[IBIS Ver]   3.2
[File Name]   sprm144.ibs
[File Rev]   0.3
[Date]   March 17, 2003
[Source]   IBIS Model Generated from PACED 4.51D
[Disclaimer]   Please be aware that in the absence of a written agreement
|   Texas Instruments(TI) assumes no liability for:
|   (1) The accuracy of the IBIS models provided to your company
|   (2) The proper functioning of these Models in your design
|   or for any resulting applications; or
|   (3)Infringement of patents, copyrights or intellectual
|   property rights resulting from your use of these models.
|   TI provides IBIS Models as a service to our customers and
|   therefore reserves the right to limit distribution of the
|   Models.
[Copyright]   Property of Texas Instruments Incorporated.
|   Unauthorized reproduction and/or distribution is strictly.
|   prohibited.
|   This product is protected under copyright law and trade
|   secret law as an unpublished work.
|   Created 2002,(C) Copyright 2002,
|   Texas Instruments Incorporated., All Rights Reserved.
|   These commodities are under the U.S.
|   Government distribution license control. As such,they are
|   not to be re-exported without the prior approval of the U.S.
|   Department of Commerce.
[Notes]   Revision History
|   0.3  Updated CLKOUT3 buffer to reflect silicon revision 2.0
|   for C6712D GDP device.
[Component]   c6712d_GDP
[Manufacturer]   Texas Instruments
[Package]
| Variable   Typ   Min   Max
R_pkg   0.15798   0.1249   0.19129
L_pkg   4.816e-09   3.586e-09   6.029e-09
C_pkg   1.362e-12   8.298e-13   1.789e-12
[Pin] signal_name   model_name   R_pin   L_pin   C_pin
A3   CLKIN   IDH091PE1001   0.18019   5.664E-09   1.7625E-12
Y12   CLKOUT2/GP2   IDH091UOS335PE1001  0.16709   5.124E-09   1.4203E-12
D10   CLKOUT3   OUK831PE1001   0.12485   3.586E-09   9.165E-13
C4   CLKMODE0   IDH091PS1001   0.15399   4.656E-09   1.3457E-12
B7   TMS   IDH091PS1001   0.15672   4.757E-09   1.3298E-12
A8   TDO   OUK831PS1001   0.16876   5.201E-09   1.4526E-12
A7   TDI   IDH091PS1001   0.17187   5.326E-09   1.4901E-12
A6   TCK   IDH091PS1001   0.17452   5.436E-09   1.563E-12
B6   TRSTz   IDH091PE1001   0.15745   4.805E-09   1.3514E-12
B12   EMU5   IDH091OUK831PS1001  0.1503   4.526E-09   1.2197E-12
C11   EMU4   IDH091OUK831PS1001  0.13457   3.948E-09   1.034E-12
B10   EMU3   IDH091OUK831PS1001  0.14073   4.347E-09   1.3521E-12
D3   EMU2   IDH091OUK831PS1001  0.15496   4.735E-09   1.2636E-12
B9   EMU1   IDH091OUK831PS1001  0.15386   4.643E-09   1.2548E-12
D9   EMU0   IDH091OUK831PS1001  0.12688   3.663E-09   9.161E-13
A13   RESETz   IDG091PS1001   0.1637   5.019E-09   1.3754E-12
C13   NMI   IDH091PE1001   0.139   4.115E-09   1.1233E-12
E3   GP7   IDH091OUK831PS1001  0.14773   4.469E-09   1.2867E-12
D2   GP6   IDH091OUK831PS1001  0.16895   5.218E-09   1.4683E-12
C1   GP5   IDH091OUK831PS1001  0.17903   5.639E-09   1.7233E-12
C2   GP4   IDH091OUK831PS1001  0.15766   4.795E-09   1.383E-12
V6   CE3z   IDH091OUK831PS1001  0.14621   4.39E-09   1.2151E-12
W6   CE2z   IDH091OUK831PS1001  0.16098   4.921E-09   1.4132E-12
W18   CE1z   IDH091OUK831PS1001  0.17556   5.446E-09   1.6489E-12
V17   CE0z   IDH091OUK831PS1001  0.15744   4.8E-09   1.3798E-12
U19   BE1z   IDH091OUK831PS1001  0.16093   4.997E-09   1.4815E-12
V20   BE0z   IDH091OUK831PS1001  0.17611   5.497E-09   1.6313E-12
J18   HOLDAz   IDH091OUK831PS1001  0.14188   4.206E-09   1.1141E-12
J17   HOLDz   IDH091OUK831PS1001  0.13083   3.807E-09   9.644E-13
J19   BUSREQ   IDH091OUK831PS1001  0.14582   4.359E-09   1.1679E-12
Y11   ECLKIN   IDH091PE1001   0.16208   0.000000005   1.4122E-12
Y10   ECLKOUT   UOS335PE1001   0.16106   4.931E-09   1.345E-12
V11   SDCASz   IDH091OUK831PS1001  0.1364   4.059E-09   1.03E-12
W10   SDRASz   IDH091OUK831PS1001  0.1486   4.45E-09   1.1911E-12
V12   SDWEz   IDH091OUK831PS1001  0.14012   4.139E-09   1.0969E-12
Y5   ARDY   IDH091OUK831PS1001  0.17592   5.451E-09   1.6354E-12
U18   EA21   IDH091OUK831PS1001  0.13802   4.156E-09   1.129E-12
Y18   EA20   IDH091OUK831PS1001  0.18588   5.849E-09   1.7404E-12
W17   EA19   IDH091OUK831PS1001  0.16927   5.225E-09   1.5492E-12
Y16   EA18   IDH091OUK831PS1001  0.17911   5.584E-09   1.6036E-12
V16   EA17   IDH091OUK831PS1001  0.15217   4.613E-09   1.3114E-12
Y15   EA16   IDH091OUK831PS1001  0.17574   5.447E-09   1.5678E-12
W15   EA15   IDH091OUK831PS1001  0.16072   4.894E-09   1.4026E-12
Y14   EA14   IDH091OUK831PS1001  0.1722   5.313E-09   1.5193E-12
W14   EA13   IDH091OUK831PS1001  0.15855   4.806E-09   1.3767E-12
V14   EA12   IDH091OUK831PS1001  0.14298   4.247E-09   1.1833E-12
W13   EA11   IDH091OUK831PS1001  0.15509   4.674E-09   1.3133E-12
V10   EA10   IDH091OUK831PS1001  0.1353   3.969E-09   1.0187E-12
Y9   EA9   IDH091OUK831PS1001  0.1646   5.033E-09   1.4055E-12
V9   EA8   IDH091OUK831PS1001  0.13792   4.071E-09   1.0499E-12
Y8   EA7   IDH091OUK831PS1001  0.16615   5.125E-09   1.4253E-12
W8   EA6   IDH091OUK831PS1001  0.1525   4.599E-09   1.2789E-12
V8   EA5   IDH091OUK831PS1001  0.14065   4.164E-09   1.1235E-12
W7   EA4   IDH091OUK831PS1001  0.15712   4.787E-09   1.3445E-12
V7   EA3   IDH091OUK831PS1001  0.1433   4.261E-09   1.1748E-12
Y6   EA2   IDH091OUK831PS1001  0.17352   5.39E-09   1.5923E-12
T19   ED15   IDH091OUK831PS1001  0.16189   4.967E-09   1.4499E-12
T20   ED14   IDH091OUK831PS1001  0.17215   5.387E-09   1.5831E-12
T18   ED13   IDH091OUK831PS1001  0.15033   4.53E-09   1.3312E-12
R20   ED12   IDH091OUK831PS1001  0.17084   5.33E-09   1.5388E-12
R19   ED11   IDH091OUK831PS1001  0.15882   4.87E-09   1.3707E-12
P20   ED10   IDH091OUK831PS1001  0.16585   5.138E-09   1.4498E-12
P18   ED9   IDH091OUK831PS1001  0.14348   4.278E-09   1.1512E-12
N20   ED8   IDH091OUK831PS1001  0.16474   5.075E-09   1.4344E-12
N19   ED7   IDH091OUK831PS1001  0.15249   4.606E-09   1.2735E-12
N18   ED6   IDH091OUK831PS1001  0.1392   4.109E-09   1.0975E-12
M20   ED5   IDH091OUK831PS1001  0.16351   4.995E-09   1.4105E-12
M19   ED4   IDH091OUK831PS1001  0.15158   4.535E-09   1.2513E-12
L19   ED3   IDH091OUK831PS1001  0.15121   4.529E-09   1.2368E-12
L18   ED2   IDH091OUK831PS1001  0.13524   3.962E-09   1.023E-12
K19   ED1   IDH091OUK831PS1001  0.14992   4.542E-09   1.2211E-12
K18   ED0   IDH091OUK831PS1001  0.13736   4.069E-09   1.0426E-12
F1   TOUT1   IDH091OUK831PE1001  0.17453   5.437E-09   1.5615E-12
F2   TINP1   IDH091OUK831PE1001  0.15861   4.866E-09   1.3778E-12
G1   TOUT0   IDH091OUK831PE1001  0.16999   5.241E-09   1.5004E-12
G2   TINP0   IDH091OUK831PE1001  0.15603   4.739E-09   1.3418E-12
E1   CLKS1   IDG091UOS205   0.17483   5.458E-09   1.617E-12
M1   CLKR1   IDH091OUK831PE1001  0.16737   5.138E-09   1.4594E-12
L3   CLKX1   IDH091OUK831PE1001  0.13844   4.083E-09   1.0869E-12
M2   DR1   IDG091UOS205   0.15325   4.608E-09   1.3011E-12
L2   DX1   IDH091OUK831PS1001  0.15147   4.517E-09   1.3075E-12
M3   FSR1   IDH091OUK831PE1001  0.13992   4.134E-09   1.1163E-12
L1   FSX1   IDH091OUK831PE1001  0.16353   4.946E-09   1.4648E-12
K3   CLKS0   IDH091OUK831PE1001  0.13597   4.005E-09   1.0142E-12
H3   CLKR0   IDH091OUK831PE1001  0.13887   4.103E-09   1.1188E-12
G3   CLKX0   IDH091OUK831PE1001  0.14227   4.232E-09   1.1737E-12
J1   DR0   IDH091OUK831PS1001  0.16689   5.141E-09   1.3597E-12
H2   DX0   IDH091OUK831PS1001  0.15223   4.578E-09   1.31E-12
J3   FSR0   IDH091OUK831PE1001  0.13605   4.002E-09   1.0327E-12
H1   FSX0   IDH091OUK831PE1001  0.16688   5.126E-09   1.4562E-12
| End of package information
| Component   IDG091PS1001
[Component]   IDG091PS1001
[Manufacturer]   Texas Instruments
[Package]
|   typ   min   max
R_pkg   0   0   0
L_pkg   0   0   0
C_pkg   0   0   0
[Pin]   signal_name   model_name   R_pin   L_pin   C_pin
   1   A   IDG091PS1001   0   0   0
| Component   IDG091UOS205
[Component]   IDG091UOS205
[Manufacturer]   Texas Instruments
[Package]
|   typ   min   max
R_pkg   0   0   0
L_pkg   0   0   0
C_pkg   0   0   0
[Pin]   signal_name   model_name   R_pin   L_pin   C_pin
   1   Y   IDG091UOS205   0   0   0
| Component   IDH091OUK831PE1001
[Component]   IDH091OUK831PE1001
[Manufacturer]   Texas Instruments
[Package]
|   typ   min   max
R_pkg   0   0   0
L_pkg   0   0   0
C_pkg   0   0   0
[Pin]   signal_name   model_name   R_pin   L_pin   C_pin
   1   Y  IDH091OUK831PE1001   0   0   0
| Component   IDH091OUK831PS1001
[Component]   IDH091OUK831PS1001
[Manufacturer]   Texas Instruments
[Package]
|   typ   min   max
R_pkg   0   0   0
L_pkg   0   0   0
C_pkg   0   0   0
[Pin]   signal_name   model_name   R_pin   L_pin   C_pin
   1   Y  IDH091OUK831PS1001   0   0   0
| Component   IDH091PE1001
[Component]   IDH091PE1001
[Manufacturer]   Texas Instruments
[Package]
|   typ   min   max
R_pkg   0   0   0
L_pkg   0   0   0
C_pkg   0   0   0
[Pin]   signal_name   model_name   R_pin   L_pin   C_pin
   1   A   IDH091PE1001   0   0   0
| Component   IDH091PS1001
[Component]   IDH091PS1001
[Manufacturer]   Texas Instruments
[Package]
|   typ   min   max
R_pkg   0   0   0
L_pkg   0   0   0
C_pkg   0   0   0
[Pin]   signal_name   model_name   R_pin   L_pin   C_pin
   1   A   IDH091PS1001   0   0   0
| Component   IDH091UOS335PE1001
[Component]   IDH091UOS335PE1001
[Manufacturer]   Texas Instruments
[Package]
|   typ   min   max
R_pkg   0   0   0
L_pkg   0   0   0
C_pkg   0   0   0
[Pin]   signal_name   model_name   R_pin   L_pin   C_pin
   1   Y  IDH091UOS335PE1001   0   0   0
| Component   OUK831PS1001
[Component]   OUK831PS1001
[Manufacturer]   Texas Instruments
[Package]
|   typ   min   max
R_pkg   0   0   0
L_pkg   0   0   0
C_pkg   0   0   0
[Pin]   signal_name   model_name   R_pin   L_pin   C_pin
   1   Y   OUK831PS1001   0   0   0
| Component   UOS335PE1001
[Component]   UOS335PE1001
[Manufacturer]   Texas Instruments
[Package]
|   typ   min   max
R_pkg   0   0   0
L_pkg   0   0   0
C_pkg   0   0   0
[Pin]   signal_name   model_name   R_pin   L_pin   C_pin
   1   Y   UOS335PE1001   0   0   0
| Models and submodels in the file (9): IDG091PS1001 (Input), IDG091UOS205 (I/O_open_drain), IDH091OUK831PE1001 (I/O), IDH091OUK831PS1001 (I/O), IDH091PE1001 (Input), IDH091PS1001 (Input), IDH091UOS335PE1001 (I/O), OUK831PS1001 (3-state), UOS335PE1001 (3-state)
